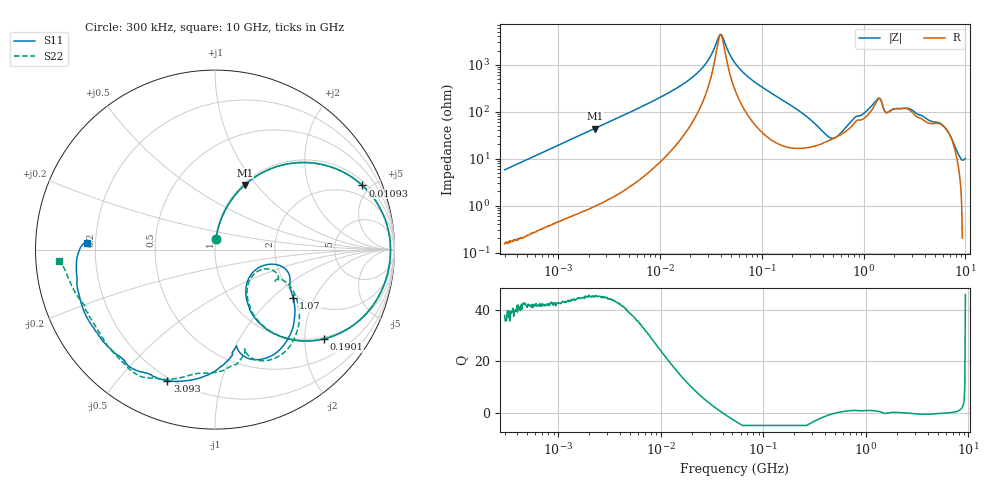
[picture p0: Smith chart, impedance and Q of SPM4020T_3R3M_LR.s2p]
! S-Parameter Data Generated by TDK Corporation
! Copyright(C) 2019 TDK Corporation.
! All Rights Reserved.
! TDK P/N: SPM4020T-3R3M-LR (Inductor)
! Property: L=3.3uH at 100kHz
! Size(LxWxT): 4.4x4.1x2mm
! Model Type: s2p (Touchstone File Format Version 1.0)
! Frequency: DC=Yes Start=0.3MHz Stop=10000MHz 802points Log-sweep
! Model Generated on Sep. 23, 2019
! Port Assignments:
!  1 ---@@@--- 2
! Applicable Conditions:
!  Temperature = 25 degC
!  DC Bias Current = 0 A
!  Small Signal Operation
! Terms and conditions regarding TDK Simulation Models
! (1)This simulation model is being provided solely for informational purposes. Please refer to the specifications of the products in terms of detailed characteristics of such products.
! (2)In no event shall TDK Corporation of any of its subsidiaries be liable for any loss or damage arising, directly or indirectly,
!  From any information contained in this simulation model, including, but not limited to loss or damages arising from any inaccuracies, omissions or errors in connection with such information.
! (3)Any and all copyrights on this simulation model are owned by TDK Corporation.
!  Duplication or redistribution of this simulation model without prior written permission from TDK Corporation is prohibited.
! (4)This simulation model is subject to any modification or change without any prior notice.
! (5)Neither TDK Corporation nor any of its subsidiaries shall make any warranty, express or implied,
!  Including but not limited to the correctness, implied warranties of merchantability and fitness for a particular purpose with respect to this simulation models.
! (6)The use of this simulation model shall be deemed to have consented to the terms and conditions hereof.
# Hz S MA R 50
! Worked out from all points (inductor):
!   801 points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, 300 kHz to 10 GHz, reference 50 ohm
!   read as one part in series: L = 3.05 uH near 318.3 kHz
!   highest Q = 45.3 at 2.308 MHz (marker M1), where L = 3.01 uH
!   self-resonance near 39.64 MHz
!   S11 on the Smith chart (normalised r, x): 300 kHz: 1.00, +0.11; 10.93 MHz: 1.24, +4.47; 190.1 MHz: 0.96, -2.48; 1.07 GHz: 1.89, -1.38; 3.093 GHz: 0.19, -0.68; 10 GHz: 0.17, +0.03
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300000  0.05717 85.1  0.9969 -3.3  0.9968 -3.3  0.05698 85.2
1713600  0.3062 70.8  0.9451 -17.9  0.9451 -17.9  0.3062 70.8
2308121  0.3962 65.3  0.9095 -23.4  0.9095 -23.4  0.3962 65.3
4982740  0.6786 45.6  0.7172 -42.9  0.7172 -42.9  0.6786 45.6
9671944  0.8723 26.7  0.4551 -61.0  0.4552 -61.0  0.8722 26.7
1.092564e7  0.8954 23.5  0.4064 -63.9  0.4064 -63.9  0.8954 23.5
2.504582e7  0.9718 6.2  0.1262 -74.5  0.1262 -74.5  0.9718 6.2
3.904515e7  0.9778 -1.3  0.0225 -11.4  0.0225 -11.5  0.9779 -1.2
5.477226e7  0.9724 -7.1  0.08942 67.5  0.08944 67.5  0.9724 -7.0
8.857507e7  0.9453 -16.7  0.2323 66.4  0.2323 66.4  0.9453 -16.7
1.900804e8  0.7848 -39.3  0.535 44.0  0.535 44.0  0.7848 -39.3
3.126428e8  0.5344 -56.7  0.724 19.3  0.7241 19.3  0.5348 -56.5
5.745924e8  0.2445 -35.1  0.7521 -17.6  0.7522 -17.6  0.255 -34.8
7.726947e8  0.3496 -13.8  0.6386 -36.6  0.6387 -36.7  0.3625 -20.6
1.069912e9  0.5118 -31.6  0.5059 -51.4  0.5059 -51.4  0.472 -26.4
1.418928e9  0.6676 -58.6  0.2805 -49.6  0.2806 -49.6  0.684 -53.3
1.767019e9  0.5496 -77.4  0.383 -50.6  0.3831 -50.6  0.5815 -73.3
2.294622e9  0.6538 -87.3  0.3008 -60.9  0.3009 -61.0  0.689 -92.9
3.093017e9  0.7773 -110.0  0.2461 -59.6  0.2461 -59.7  0.7691 -110.1
6.253087e9  0.8054 -139.1  0.2111 -92.3  0.2113 -92.4  0.7968 -142.2
8.09931e9  0.794 -165.8  0.1784 -115.5  0.1785 -115.6  0.8247 -166.3
1e10  0.7145 177.0  0.1345 -126.2  0.1345 -126.3  0.8709 -175.9
